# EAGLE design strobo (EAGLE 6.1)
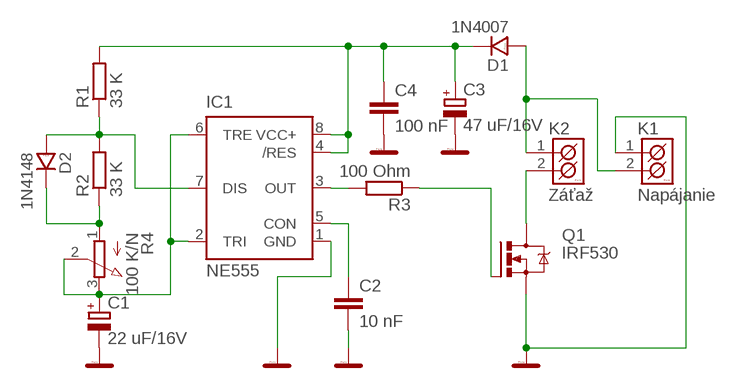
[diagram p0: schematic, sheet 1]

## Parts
C1  22 uF/16V  CPOL-EUE2.5-6  [E2,5-6]
C2  10 nF  C-EU050-030X075  [C050-030X075]
C3  47 uF/16V  CPOL-EUE2.5-6  [E2,5-6]
C4  100 nF  C-EU050-030X075  [C050-030X075]
D1  1N4007  1N4007_10  [DO41]
D2  1N4148  1N4148_7,5  [DO35]
IC1  NE555  [DIL-08]
K1  Napájanie  ARK500/2  [ARK500/2]
K2  Záťaž  ARK500/2  [ARK500/2]
Q1  IRF530  [TO220BV]
R1  33 K  R-EU_0207/10  [0207/10]
R2  33 K  R-EU_0207/10  [0207/10]
R3  100 Ohm  R-EU_0207/10  [0207/10]
R4  100 K/N  3RP/1610N  [3RP/1610N]

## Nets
GND: C1.- C2.2 C3.- C4.2 IC1.1(GND) K1.1(K1) Q1.S
N$1: D2.A IC1.7(DIS) R1.1 R2.2
N$3: D2.K R2.1 R4.1(A)
N$6: C3.+ C4.1 D1.K IC1.4(/RES) IC1.8(VCC+) R1.2
N$7: IC1.3(OUT) R3.2
N$8: Q1.G R3.1
N$9: K2.2(K2) Q1.D
N$10: D1.A K1.2(K2) K2.1(K1)
N$12: C2.1 IC1.5(CON)
N$13: C1.+ IC1.2(TRI) IC1.6(TRE) R4.2(S) R4.3(E)

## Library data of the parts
C1 C3 = resistor:CPOL-EU: POLARIZED CAPACITOR, European symbol
C2 C4 = resistor:C-EU: CAPACITOR, European symbol
D1 = #PaJa_22:1N4007: Usmernovaci dioda - 1A, 1000V
D2 = #PaJa_22:1N4148: Univerzalni dioda - 0,15A, 75V
IC1 = st-microelectronics:NE555: General purpose bipolar Timer; MF: Arrow Electronics; MPN: NE555N; OC_FARNELL: 1467742; OC_NEWARK: 89K1486
K1 K2 = #PaJa_konektory:ARK500/2: Svorkovnice - roztec 5mm - dvojita
Q1 = transistor-power:IRF530: HEXFET Power MOSFET
R1-R3 = resistor:R-EU_: RESISTOR, European symbol
R4 = pot:3RP/1610N: 16mm Potentiometer one level Source: http://www.alphapotentiometers.net/html/16mm_pot_2.html

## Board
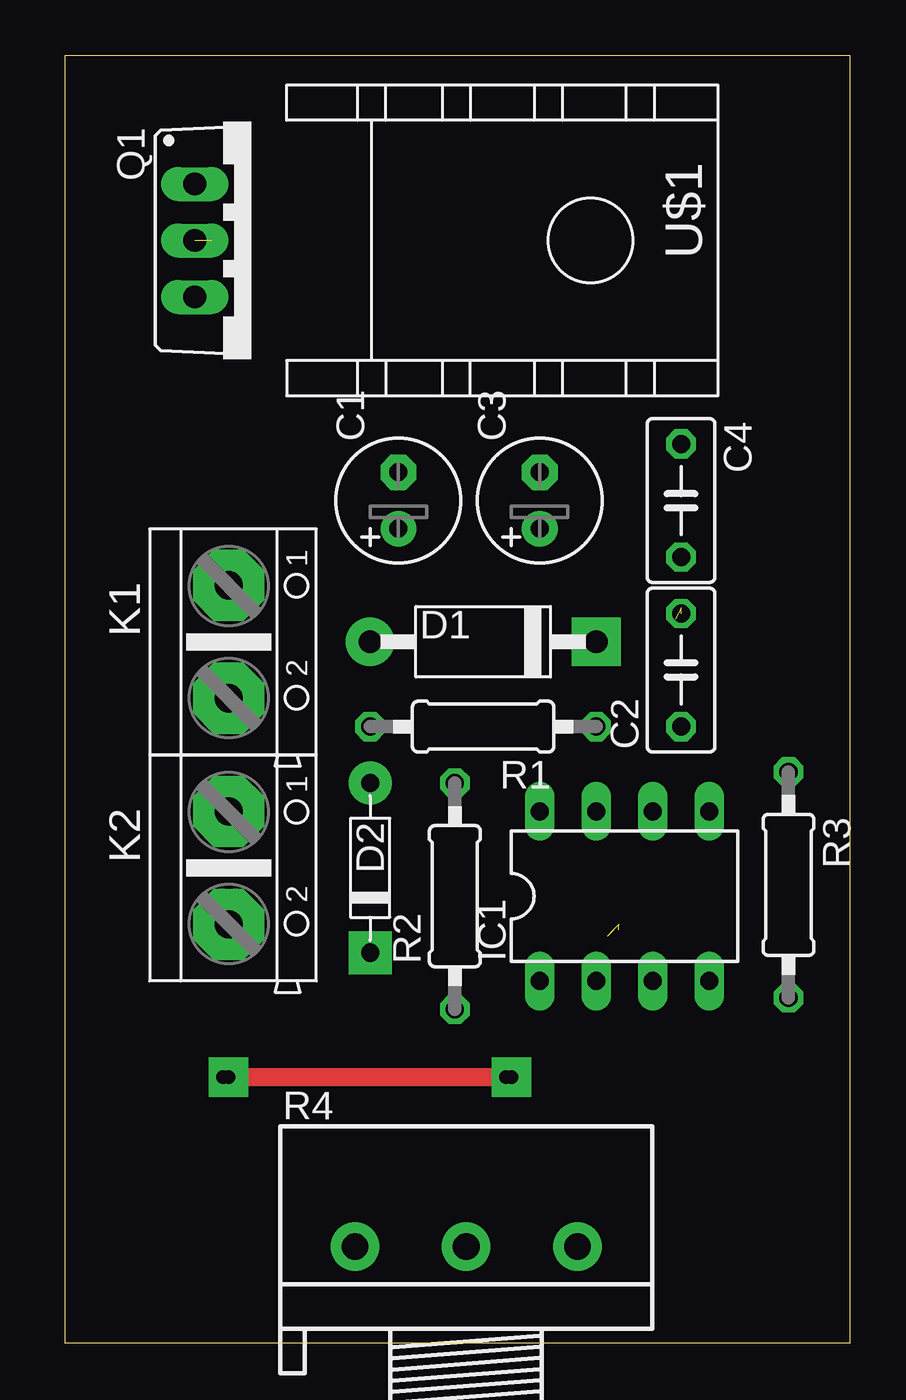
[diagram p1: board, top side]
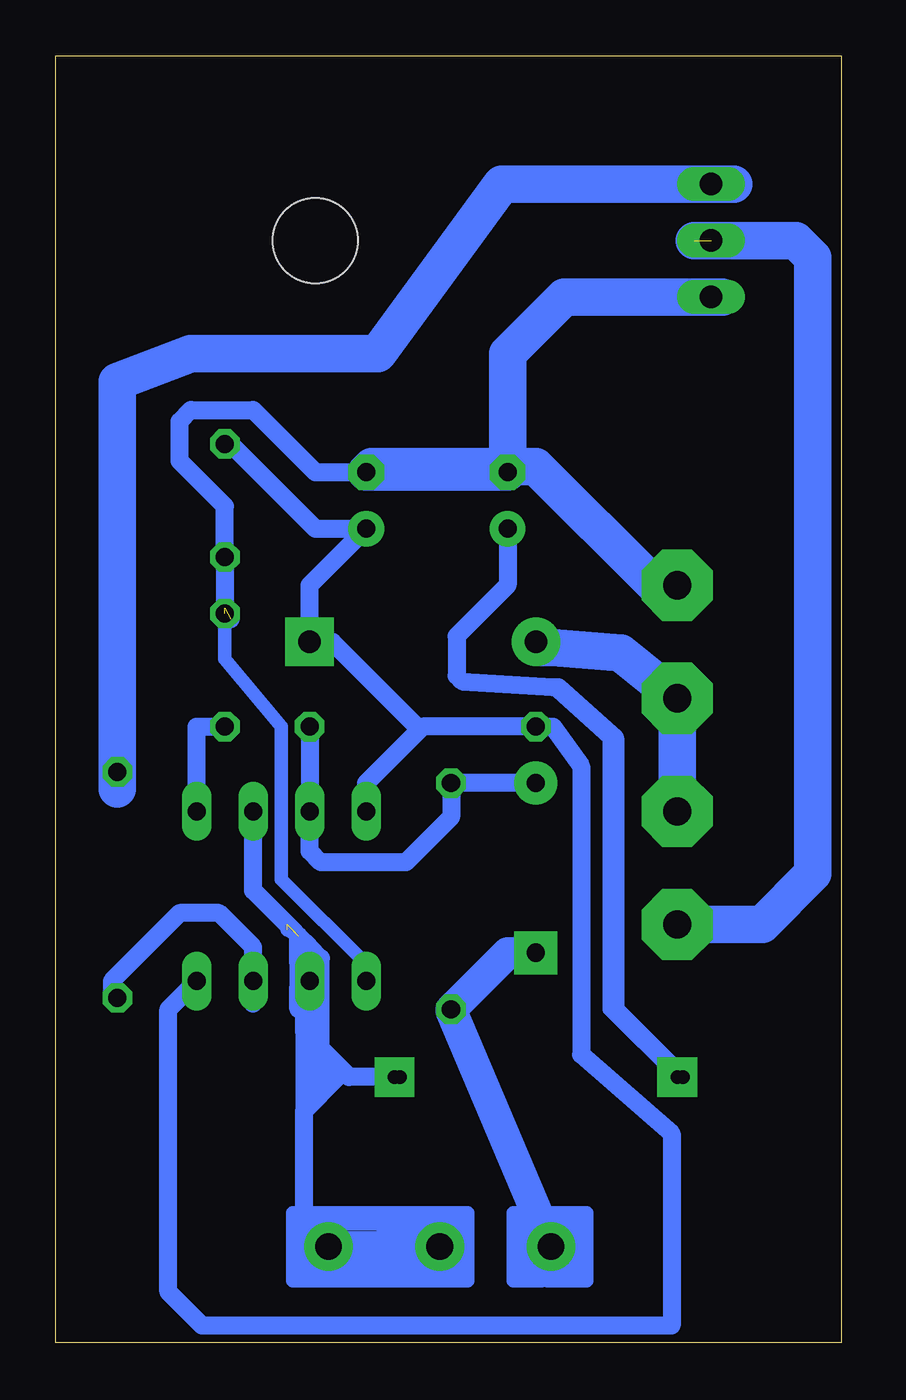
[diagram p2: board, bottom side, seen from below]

Size 35.29 x 57.84 mm. Coordinates in mm from the lower left corner, seen from the top.
Outline: 0,0 35.29,0 35.29,57.84 0,57.84 0,0
Copper layers (1*16): Top 0.035mm / dielectric 1.5mm / Bottom 0.035mm
Design rules: minimum track width 10mil, minimum drill 24mil, track to track 8mil, track to pad 8mil, pad to pad 8mil, via to via 8mil, smd to smd 8mil, copper to edge 40mil, drill to drill 8mil, minimum pad ring 10mil, minimum via ring 8mil, stop-mask expansion 4mil, vias tented up to drill 0mil, thermal gap 10mil

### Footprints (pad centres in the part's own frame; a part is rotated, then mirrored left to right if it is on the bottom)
E2,5-6 = drill 0.813 pad 1.6: + -1.27,0 | drill 0.813 pad 1.6 octagon: - 1.27,0
C050-030X075 = drill 0.813 octagon: 1 -2.54,0; 2 2.54,0
DO41 = drill 1.016 pad 2.184: A -5.08,0 | drill 1.016 pad 2.184 square: K 5.08,0
DO35 = drill 0.813 pad 1.93: A -3.81,0 | drill 0.813 pad 1.93 square: K 3.81,0
DIL-08 = drill 0.813 long: 1 -3.81,-3.81; 2 -1.27,-3.81; 3 1.27,-3.81; 4 3.81,-3.81; 5 3.81,3.81; 6 1.27,3.81; 7 -1.27,3.81; 8 -3.81,3.81
ARK500/2 = drill 1.27 pad 3.2 octagon: 1 -2.54,0; 2 2.54,0
TO220BV = drill 1.016 long: D 0,-2.54; G -2.54,-2.54; S 2.54,-2.54
0207/10 = drill 0.813 octagon: 1 -5.08,0; 2 5.08,0
3RP/1610N = drill 1.2 pad 2.184: 1 -5,0; 2 0,0; 3 5,0
CH_DO1-3 = hole 3.81: 0,0

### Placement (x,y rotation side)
C1  14.99,37.85 90 top
C2  27.69,30.23 90 top
C3  21.34,37.85 90 top
C4  27.69,37.85 270 top
D1  18.8,31.5 0 top
D2  13.72,21.34 270 top
IC1  25.15,20.07 0 top
K1  7.37,31.5 270 top
K2  7.37,21.34 270 top
Q1  8.38,49.53 270 top
R1  18.8,27.69 180 top
R2  17.53,20.07 90 top
R3  32.51,20.57 270 top
R4  18.03,4.32 0 top
U$1  [CH_DO1-3]  23.62,49.53 270 top

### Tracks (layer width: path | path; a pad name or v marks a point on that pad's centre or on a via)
GND  (2 unrouted)
  Bottom 0.61: IC1.1 21.34,17.02 25.15,20.83 25.15,27.69 27.69,30.73 C2.2
  Bottom 0.813: C3.- 23.62,39.12 26.42,41.91 29.21,41.91 29.72,41.4 29.72,39.62 27.69,37.59 C4.2 C2.2 27.43,32.77 27.43,32.51 | IC1.1 21.08,16.26 21.08,16 21.34,16 IC1.1
  Bottom 1.016: C1.- C3.-
  Bottom 1.676: 21.08,39.37 21.08,39.12 C1.- 14.99,44.45 12.45,46.99 Q1.S 5.33,46.99 | K1.1 8.38,34.04 13.72,39.37 21.08,39.37 | 21.08,39.37 C3.-
N$1
  Bottom 0.813: D2.A R2.2 17.53,23.62 19.56,21.59 23.37,21.59 23.88,22.1 IC1.7 R1.1
N$3
  Bottom 1.422: D2.K 14.99,17.53 R2.1 17.53,14.91 R4.1
N$4  (via drill 0.6)
  other vias: 19.81,11.94
N$6
  Bottom 0.813: C4.1 27.43,40.39 23.62,36.58 C3.+ 23.88,34.04 D1.K 22.86,31.5 18.92,27.56 | 18.92,27.56 18.8,27.69 R1.2 12.95,27.69 11.68,25.91 11.68,12.95 7.62,9.4 7.62,0.76 28.7,0.76 30.23,2.29 30.23,14.99 IC1.4 | IC1.8 21.34,25.15 18.92,27.56
N$7
  Bottom 0.813: 26.42,15.24 IC1.3 26.42,17.78 27.94,19.3 29.72,19.3 32.77,16.26 32.77,15.75 R3.2
N$8
  Bottom 1.676: 32.51,24.89 R3.1 32.51,43.18 29.21,44.45 20.83,44.45 15.24,52.07 Q1.G 4.83,52.07
N$9  (1 unrouted)
  Bottom 1.676: K2.2 3.56,18.8 1.27,21.08 1.27,48.77 2.03,49.53 6.6,49.53
N$10
  Bottom 1.676: K2.1 K1.2 9.91,30.99 12.95,31.24 13.46,31.24 D1.A
N$11
  Bottom 0.61: 13.21,4.06 13.21,2.79 11.43,2.79 11.43,5.84 14.73,5.84 14.73,3.05 | 14.22,3.05 13.46,3.05 | 11.68,3.05 13.46,3.05 | 13.46,3.05 13.46,2.79 14.73,2.79 14.73,3.05 | 14.73,3.05 14.22,3.05 | 14.22,3.05 14.22,5.33 13.97,5.33 13.97,3.3 11.94,3.3 11.94,5.33 | 11.94,5.33 12.7,5.33 | 11.94,5.33 11.68,5.33 11.68,3.3
N$12
  Bottom 0.813: IC1.5 28.96,27.69 C2.1
N$13  (via drill 0.6, 0.6 pad 1.78)  (4 unrouted)
  Top 0.813: v7.11,11.94 v7.37,11.94 v19.81,11.94
  Bottom 0.61: 16.76,3.56 16.76,5.84 19.56,5.84 | 19.56,5.84 19.56,3.05 | 16.76,3.05 16.76,2.79 19.56,2.79 | 19.56,3.05 16.76,3.05 | 16.76,3.05 16.76,3.56 | 16.76,3.56 17.02,3.56 17.02,5.33 19.05,5.33 19.05,3.3 17.02,3.3 | 19.56,5.84 24.64,5.84 24.64,2.79 19.56,2.79 | 19.56,2.79 19.56,3.05 | 19.56,3.05 20.07,3.05 20.07,5.33 20.57,5.33 | 20.57,5.33 20.57,3.3 21.08,3.3 21.08,4.06 | 12.95,29.46 10.41,27.18 10.41,14.99 v7.37,11.94 7.11,11.68 | v20.07,11.94 22.61,11.94 | 23.37,12.7 23.37,16 23.88,16.51 | 24.64,18.54 24.89,18.54 | 20.57,5.33 24.13,5.33 24.13,3.3 23.88,3.3 | 23.88,3.3 21.59,3.3 | 21.59,3.3 21.59,3.56 23.88,3.56 23.88,3.3 | 21.59,3.3 21.34,3.3 21.34,4.32
  Bottom 0.813: C1.+ 14.99,34.04 17.27,31.75 17.27,29.97 17.02,29.72 12.95,29.46 12.7,29.46 10.16,27.18 10.16,14.99 v7.11,11.94 | R4.2 21.08,4.06 24.13,4.06 24.13,10.41 | 24.13,13.97 24.13,16 IC1.2 | IC1.2 23.62,16.51 23.88,16.51 | v19.81,11.94 v20.07,11.94 22.1,11.94 24.13,13.97 | 24.13,13.97 24.13,10.41 | 24.13,10.41 22.61,11.94 23.37,12.7 | 23.37,12.7 23.88,13.21 23.88,11.94 23.62,11.94 23.37,11.68 23.37,12.7 | 23.37,12.7 23.37,17.27 23.88,17.78 | 23.88,16 IC1.2 | IC1.2 23.88,16.51 | 23.88,16.51 24.38,17.02 | 24.38,17.02 24.38,17.53 | 24.13,17.78 24.38,17.53 | 24.38,17.53 24.38,18.29 | 24.38,17.02 24.38,16 | 24.38,14.99 24.38,16 | 24.38,16 23.88,16.51 | 23.88,16.51 23.88,17.78 | 24.38,18.29 24.64,18.54 26.42,20.32 IC1.6 | 23.88,17.78 24.38,18.29
  Bottom 1.422: R4.3 21.34,4.32 R4.2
